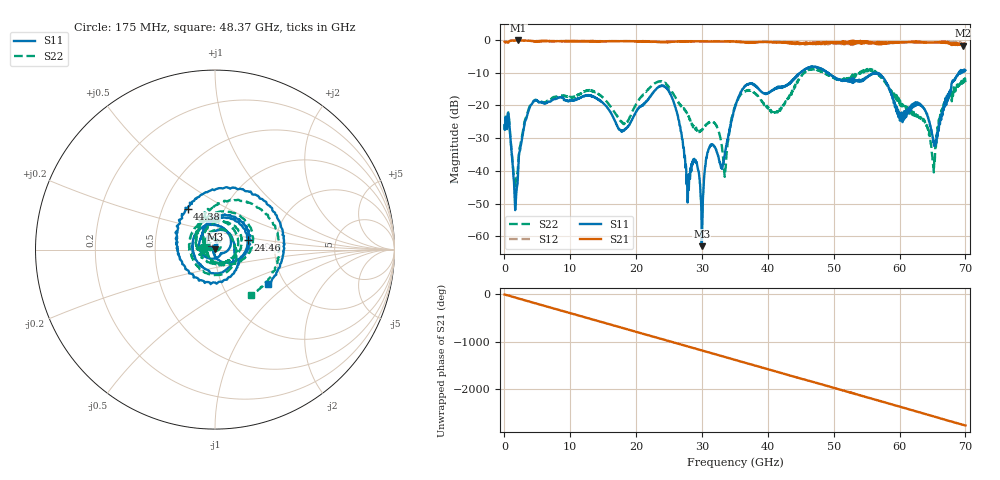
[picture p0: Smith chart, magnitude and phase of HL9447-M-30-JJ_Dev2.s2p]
! 8/12/2020 3:41:56 PM
! H:\PRODUCTION_DATA\TEMP_S2P.S2P
! CHANNEL.1
! TR.MEASUREMENT
! CORRECTED.DATA
# GHZ S RI R 50.0
! FREQ.GHZ  S11RE  S11IM  S21RE  S21IM  S12RE  S12IM  S22RE  S22IM
!; PortSelection: Port_12
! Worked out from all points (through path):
!   2000 points, 35 MHz to 70 GHz, reference 50 ohm
!   highest |S21| = -0.11 dB at 2.1 GHz (marker M1); lowest = -1.7 dB at 69.61 GHz (marker M2)
!   group delay of S21, straight-line fit = 110 ps
!   lowest |S11| = -63.0 dB at 29.96 GHz (marker M3), VSWR 1.00, Z = 50 + j0.0595 ohm
!   |S11| at or under -10 dB: start of sweep to 44.91 GHz; 49.12 GHz to 56 GHz (6.881 GHz wide, 13.1 % of centre); 56.56 GHz to 69.07 GHz (12.51 GHz wide, 19.9 % of centre)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
!   |S22| runs from -45.4 to -8.8 dB; largest |S21 - S12| = 0.15
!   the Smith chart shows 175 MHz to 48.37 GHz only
!   S11 on the Smith chart (normalised r, x): 175 MHz: 0.88, +0.02; 24.46 GHz: 1.44, +0.16; 44.38 GHz: 0.67, +0.33; 48.37 GHz: 1.64, -0.72
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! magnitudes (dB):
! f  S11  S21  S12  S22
! 35 MHz  -26.0  -0.5  -0.5  -25.9
! 175 MHz  -23.5  -0.7  -0.7  -23.4
! 1.645 GHz  -52.0  -0.1  -0.2  -44.6
! 2.1 GHz  -39.6  -0.1  -0.2  -37.9
! 4.34 GHz  -19.1  -0.3  -0.3  -18.9
! 11.72 GHz  -17.4  -0.3  -0.3  -16.1
! 17.92 GHz  -27.7  -0.3  -0.3  -25.2
! 23.38 GHz  -14.3  -0.6  -0.6  -12.7
! 24.46 GHz  -14.4  -0.6  -0.7  -13.2
! 27.82 GHz  -49.7  -0.4  -0.5  -22.5
! 29.96 GHz  -63.0  -0.4  -0.4  -27.6
! 31.15 GHz  -32.6  -0.4  -0.4  -25.2
! 33.46 GHz  -35.2  -0.4  -0.5  -41.8
! 35.03 GHz  -20.5  -0.5  -0.5  -20.1
! 44.38 GHz  -11.2  -0.7  -1.1  -13.1
! 46.69 GHz  -8.2  -1.1  -1.2  -8.9
! 48.37 GHz  -9.1  -0.9  -1.2  -9.9
! 58.34 GHz  -14.6  -0.7  -1.0  -14.6
! 65.17 GHz  -31.4  -0.7  -0.8  -39.0
! 66.64 GHz  -20.5  -0.8  -0.6  -20.1
! 69.61 GHz  -9.2  -1.7  -0.8  -12.4
! 70 GHz  -9.2  -1.3  -1.2  -12.9
